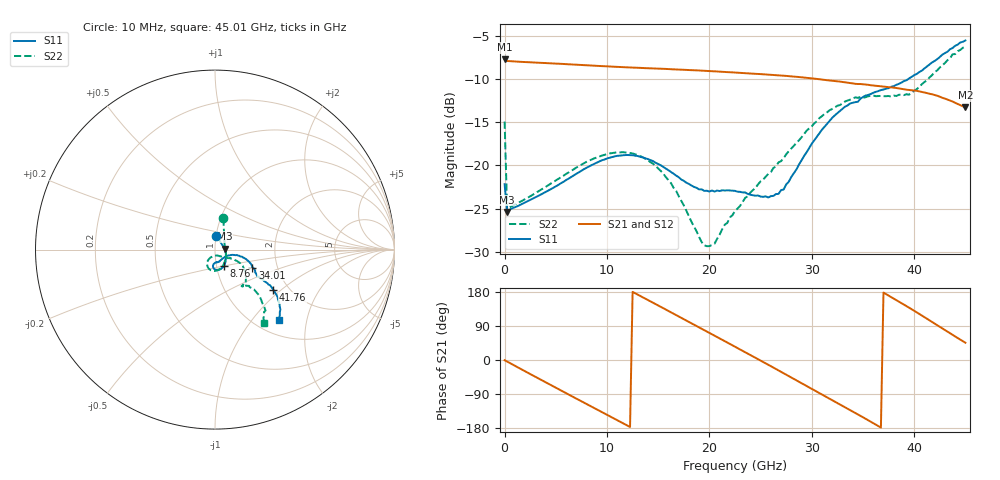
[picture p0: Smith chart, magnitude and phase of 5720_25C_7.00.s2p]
! Device:  ADRF5720
! Description: 0.5dB LSB GaAs MMIC 6-bit Digital Attenuator
! Frequency:  0.000009 -  40 GHz
! Ports:
!	RF1	= Port 1
!	RF2	= Port 2
! Vdd:  3.3 Volt
! Vss:  -3.3 Volt
! Control:  0/3.3 Volt
! State:  7.00 dB attenuation
! Data:  The device was measured using G-S-G Probes on a matrix board.
!  Data was collected using an calibrated 4 port network analyzer.
!  The reference plane for this measurement is at the launchers.
! Note:  Analog Devices supplies this data as a sample of measured data
!  for this product.  Your particular data for this product may vary.
!  Data was taken at 25 degrees C.
!  Analog Devices reserves the right to change this data at anytime.
# GHZ S DB R 45.0
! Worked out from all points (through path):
!   181 points, 10 MHz to 45.01 GHz, reference 45 ohm
!   highest |S21| = -7.71 dB at 10 MHz (marker M1); lowest = -13.3 dB at 45.01 GHz (marker M2)
!   group delay of S21, straight-line fit = 41.1 ps
!   lowest |S11| = -25.4 dB at 260 MHz (marker M3), VSWR 1.11, Z = 50.1 + j0.608 ohm
!   |S11| at or under -10 dB: start of sweep to 39.4 GHz
!   |S22| runs from -29.4 to -6.2 dB; largest |S21 - S12| = 0.00047
!   S11 on the Smith chart (normalised r, x): 10 MHz: 1.00, +0.16; 8.76 GHz: 1.09, -0.19; 34.01 GHz: 1.49, -0.31; 41.76 GHz: 1.67, -0.89; 45.01 GHz: 1.25, -1.38
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0.01  -22.18 84.7  -7.71 -0.5  -7.71 -0.5  -14.92 75.0
0.26  -25.40 6.5  -7.89 -4.0  -7.90 -4.1  -25.20 5.4
2.01  -24.29 -13.0  -8.01 -29.8  -8.01 -29.8  -23.91 -17.6
4.26  -22.92 -31.2  -8.15 -62.3  -8.15 -62.3  -22.31 -39.8
6.01  -21.70 -42.7  -8.25 -87.5  -8.25 -87.5  -20.99 -53.8
7.76  -20.43 -53.7  -8.37 -112.5  -8.37 -112.5  -19.74 -66.7
8.760001  -19.82 -60.2  -8.44 -126.8  -8.44 -126.8  -19.18 -73.8
12.01  -18.79 -81.3  -8.63 -173.1  -8.63 -173.1  -18.53 -97.8
15.26  -19.98 -95.7  -8.79 140.3  -8.79 140.3  -20.64 -118.5
17.51  -21.78 -95.6  -8.91 107.8  -8.91 107.8  -24.63 -121.7
19.51  -22.95 -86.3  -9.03 78.8  -9.03 78.8  -29.26 -94.4
20.51  -23.03 -81.1  -9.09 64.3  -9.09 64.3  -29.08 -68.3
22.76  -23.04 -71.5  -9.24 31.5  -9.25 31.5  -25.00 -42.7
24.76  -23.48 -59.1  -9.39 2.2  -9.39 2.2  -22.19 -35.0
26.76  -23.30 -36.2  -9.55 -27.4  -9.55 -27.4  -19.65 -28.3
30.26  -17.07 -14.2  -9.94 -79.8  -9.94 -79.8  -15.11 -30.5
34.01  -12.74 -25.7  -10.49 -136.2  -10.49 -136.2  -12.27 -45.0
36.01  -11.58 -30.1  -10.73 -166.6  -10.73 -166.6  -11.90 -53.2
37.76  -10.88 -32.3  -10.95 166.2  -10.96 166.3  -12.02 -53.4
39.51  -9.91 -32.4  -11.25 138.1  -11.26 138.2  -11.80 -51.3
41.76  -8.06 -34.6  -11.75 100.4  -11.75 100.4  -9.53 -45.9
45.01  -5.51 -48.1  -13.28 45.6  -13.28 45.6  -6.20 -56.2
